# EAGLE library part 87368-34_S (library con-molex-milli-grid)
RECEPTACAL
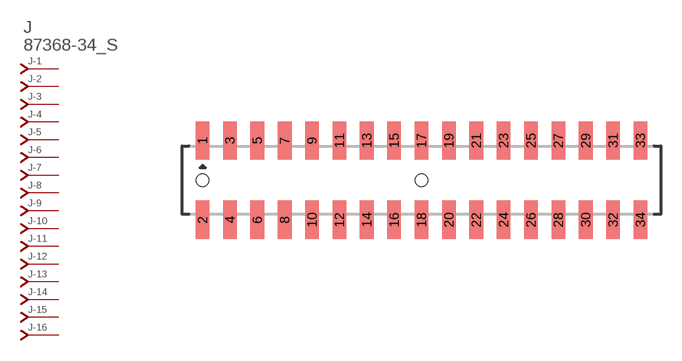
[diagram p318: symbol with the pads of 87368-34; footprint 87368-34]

Designator prefix J; gates -1=J-NV -2=J-N -3=J-N -4=J-N -5=J-N -6=J-N -7=J-N -8=J-N -9=J-N -10=J-N -11=J-N -12=J-N -13=J-N -14=J-N -15=J-N -16=J-N -17=J-N -18=J-N -19=J-N -20=J-N -21=J-N -22=J-N -23=J-N -24=J-N -25=J-N -26=J-N -27=J-N -28=J-N -29=J-N -30=J-N -31=J-N -32=J-N -33=J-N -34=J-N

## 87368-34_S  [87368-34]
1  -1:J  pas
2  -2:J  pas
3  -3:J  pas
4  -4:J  pas
5  -5:J  pas
6  -6:J  pas
7  -7:J  pas
8  -8:J  pas
9  -9:J  pas
10  -10:J  pas
11  -11:J  pas
12  -12:J  pas
13  -13:J  pas
14  -14:J  pas
15  -15:J  pas
16  -16:J  pas
17  -17:J  pas
18  -18:J  pas
19  -19:J  pas
20  -20:J  pas
21  -21:J  pas
22  -22:J  pas
23  -23:J  pas
24  -24:J  pas
25  -25:J  pas
26  -26:J  pas
27  -27:J  pas
28  -28:J  pas
29  -29:J  pas
30  -30:J  pas
31  -31:J  pas
32  -32:J  pas
33  -33:J  pas
34  -34:J  pas

## Footprint 87368-34 (pad centres in mm)
RECEPTACAL SMD Dual Row, Side Entry
smd 1 x 2.8: 1 -16,2.9; 2 -16,-2.9; 3 -14,2.9; 4 -14,-2.9; 5 -12,2.9; 6 -12,-2.9; 7 -10,2.9; 8 -10,-2.9; 9 -8,2.9; 10 -8,-2.9; 11 -6,2.9; 12 -6,-2.9; 13 -4,2.9; 14 -4,-2.9; 15 -2,2.9; 16 -2,-2.9; 17 0,2.9; 18 0,-2.9; 19 2,2.9; 20 2,-2.9; 21 4,2.9; 22 4,-2.9; 23 6,2.9; 24 6,-2.9; 25 8,2.9; 26 8,-2.9; 27 10,2.9; 28 10,-2.9; 29 12,2.9; 30 12,-2.9; 31 14,2.9; 32 14,-2.9; 33 16,2.9; 34 16,-2.9
hole 0.914 at -16,0
hole 0.914 at 0,0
